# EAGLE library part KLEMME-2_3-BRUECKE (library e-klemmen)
Klemme 3-pol. mit Brückenhinweis
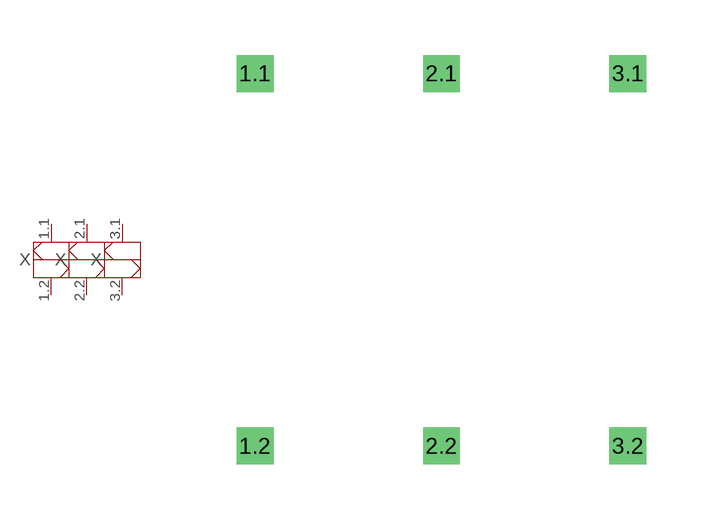
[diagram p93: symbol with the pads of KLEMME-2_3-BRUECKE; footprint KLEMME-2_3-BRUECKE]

Designator prefix X; gates 1=KLEMME-2_1-BRUECKE 2=KLEMME-2_2-BRUECKE 3=KLEMME-2_3-BRUECKE

## KLEMME-2_3-BRUECKE  [KLEMME-2_3-BRUECKE]
1.1  1:1  pas
1.2  1:2  pas
2.1  2:1  pas
2.2  2:2  pas
3.1  3:1  pas
3.2  3:2  pas

## Footprint KLEMME-2_3-BRUECKE (pad centres in mm)
Dummy
drill 0.5 pad 1 square: 1.1 0,5.08; 1.2 0,-5.08; 2.1 5.08,5.08; 2.2 5.08,-5.08; 3.1 10.16,5.08; 3.2 10.16,-5.08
